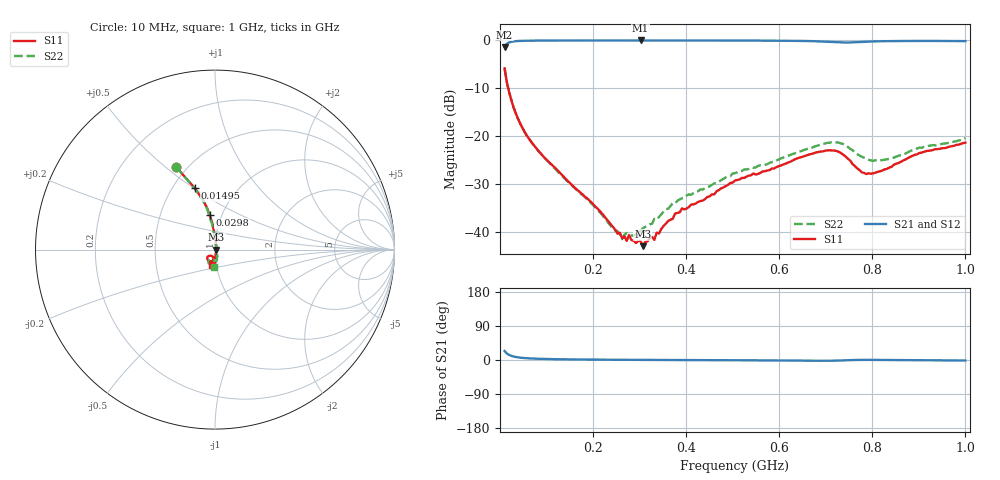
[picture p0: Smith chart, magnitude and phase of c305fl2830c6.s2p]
!Agilent Technologies,N5234A,MY52241123,A.10.00.00
!Agilent N5234A: A.10.00.00
!Date: Wednesday, September 04, 2019 09:50:15
!Correction: S11(Full 2 Port(1,2))
!S21(Full 2 Port(1,2))
!S12(Full 2 Port(1,2))
!S22(Full 2 Port(1,2))
!S2P File: Measurements: S11, S21, S12, S22:
# Hz S  dB  R 50
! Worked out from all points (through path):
!   201 points, 10 MHz to 1 GHz, reference 50 ohm
!   highest |S21| = -0.01 dB at 302.1 MHz (marker M1); lowest = -1.4 dB at 10 MHz (marker M2)
!   lowest |S11| = -43.0 dB at 307 MHz (marker M3), VSWR 1.01, Z = 50.7 - j0.0984 ohm
!   |S11| at or under -10 dB: 17.77 MHz to end of sweep
!   |S22| runs from -41.6 to -5.9 dB; largest |S21 - S12| = 0.0052
!   S11 on the Smith chart (normalised r, x): 10 MHz: 0.44, +0.54; 14.95 MHz: 0.64, +0.51; 29.8 MHz: 0.88, +0.35; 1 GHz: 0.95, -0.16
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1e7  -5.84 115.3  -1.36 23.8  -1.35 24.0  -5.88 115.2
1.495e7  -8.84 108.2  -0.67 16.9  -0.67 17.2  -8.85 108.4
2.98e7  -14.19 98.9  -0.20 9.0  -0.20 9.1  -14.14 99.5
5.455e7  -19.41 93.5  -0.07 5.0  -0.08 5.0  -19.42 94.4
7.93e7  -22.72 90.4  -0.04 3.4  -0.05 3.4  -22.79 91.4
1.783e8  -32.27 75.8  -0.02 1.2  -0.02 1.2  -32.42 74.3
2.6245e8  -41.39 29.1  -0.01 0.6  -0.02 0.6  -41.59 20.3
2.7235e8  -41.94 20.8  -0.02 0.5  -0.02 0.5  -40.28 6.5
2.773e8  -40.72 17.9  -0.01 0.4  -0.02 0.5  -40.58 1.7
2.9215e8  -42.41 6.0  -0.02 0.4  -0.02 0.4  -40.59 -15.7
2.971e8  -41.97 -0.3  -0.01 0.3  -0.01 0.4  -40.87 -15.4
3.0205e8  -42.00 -9.4  -0.01 0.3  -0.01 0.4  -39.85 -20.2
3.07e8  -43.05 -7.9  -0.01 0.3  -0.02 0.3  -39.30 -22.2
3.4165e8  -40.40 -47.4  -0.02 0.1  -0.03 0.1  -36.96 -41.5
3.9115e8  -35.16 -69.5  -0.02 -0.2  -0.02 -0.1  -33.03 -59.6
5.05e8  -29.32 -83.6  -0.03 -0.6  -0.04 -0.6  -27.77 -72.8
6.733e8  -23.65 -105.3  -0.16 -1.9  -0.17 -1.9  -22.33 -90.7
7.2775e8  -23.30 -127.9  -0.41 -1.5  -0.43 -1.5  -21.38 -110.9
7.8715e8  -27.96 -118.0  -0.27 0.4  -0.27 0.4  -24.76 -111.8
8.3665e8  -26.59 -100.3  -0.14 0.0  -0.16 0.0  -24.76 -98.3
9.01e8  -23.56 -96.7  -0.11 -0.6  -0.12 -0.5  -22.43 -91.8
1e9  -21.37 -101.2  -0.14 -1.3  -0.15 -1.3  -20.45 -93.7
